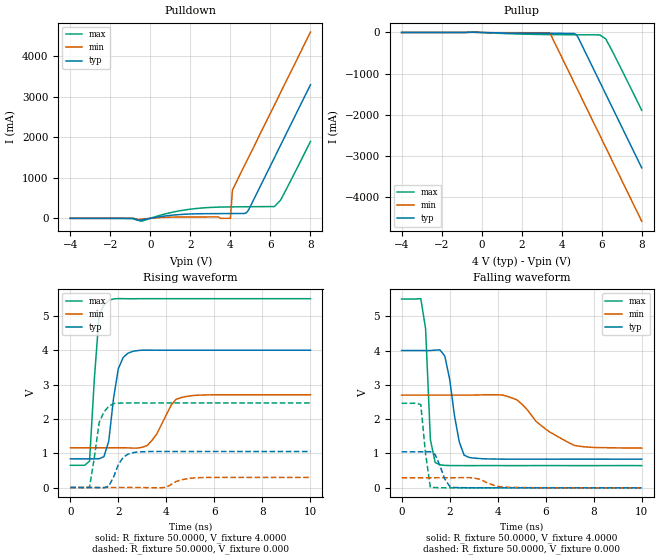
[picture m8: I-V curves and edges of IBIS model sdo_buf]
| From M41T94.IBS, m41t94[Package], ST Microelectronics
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|   Model sdo_buf
[Model]   sdo_buf
Model_type   Output
Polarity   Non-Inverting
Vmeas =   1.5000V
Cref =1.000e-10F
Rref =   0.6450k
Vref =   1.7300V
C_comp   7.8300pF   7.2500pF   8.5000pF
[Temperature Range]   27.0000   85.0000   -40.0000
[Voltage Range]   4.0000V   2.7000V   5.5000V
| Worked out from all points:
|   slope of the pulldown table from 0 to 0.6 V, typ, clamps not added: 12.4 ohm
|   slope of the pullup table from 0 to 0.6 V, typ, clamps not added: 80.2 ohm
|   rising waveform, R_fixture 50.0000, V_fixture 4.0000: 20-80 % time 359ps typ, 694ps min, 276ps max; typ from 0.835 V to 4 V
|   rising waveform, R_fixture 50.0000, V_fixture 0.000: 20-80 % time 434ps typ, 584ps min, 337ps max; typ from 0 V to 1.05 V
|   falling waveform, R_fixture 50.0000, V_fixture 4.0000: 20-80 % time 427ps typ, 1.5ns min, 180ps max; typ from 4 V to 0.835 V
|   falling waveform, R_fixture 50.0000, V_fixture 0.000: 20-80 % time 368ps typ, 636ps min, 238ps max; typ from 1.05 V to 0 V
[Pulldown]
| voltage   I(typ)   I(min)   I(max)
-4V       0A         0A         -600uA
-900mV    0A         0A         -7mA
-500mV    -45mA      -23.28mA   -72.71mA
1.6V      97.61mA    32.87mA    197mA
3.4V      116.6mA    33.89mA    276.6mA
4V        117.9mA    0A         281.9mA
4.1V      118.1mA    700mA      282.5mA
4.7V      120mA      1.3A       285.4mA
4.9V      202.4mA    1.5A       286.2mA
6.2V      1.5A       2.8A       291.2mA
6.5V      1.8A       3.1A       445.7mA
8V        3.3A       4.6A       1.899A
[Pullup]
| voltage   I(typ)   I(min)   I(max)
-4V       0A         0A         100uA
-400mV    5.701mA    2.743mA    10.5mA
3.4V      -21.56mA   -7.302mA   -51.47mA
4.6V      -23.5mA    -1.2A      -56.08mA
4.7V      -41.44mA   -1.3A      -56.35mA
4.8V      -103.4mA   -1.4A      -56.6mA
5.9V      -1.2A      -2.5A      -58.75mA
6.2V      -1.5A      -2.8A      -155.2mA
6.8V      -2.1A      -3.4A      -716.5mA
8V        -3.3A      -4.6A      -1.896A
[Ramp]
| variable   typ   min   max
dV/dt_r   2.1420/0.8210n   1.2358/2.1288n   3.1094/0.3905n
dV/dt_f   2.3600/0.2827n   1.5646/0.7749n   3.2700/0.1442n
R_load = 0.6450k
[Rising Waveform]
R_fixture = 50.0000
V_fixture = 4.0000
V_fixture_min = 2.7000
V_fixture_max = 5.5000
| time   V(typ)   V(min)   V(max)
0s        835.1mV    1.158V     647mV
800ps     835.2mV    1.158V     767.3mV
1ns       834.2mV    1.158V     3.169V
1.2ns     838.6mV    1.158V     5.023V
1.6ns     1.35V      1.158V     5.449V
2ns       3.465V     1.158V     5.503V
2.4ns     3.912V     1.155V     5.499V
3.2ns     4.002V     1.224V     5.5V
4.6ns     4V         2.617V     5.5V
10ns      4V         2.7V       5.5V
[Rising Waveform]
R_fixture = 50.0000
V_fixture = 0.000
V_fixture_min = 0.000
V_fixture_max = 0.000
| time   V(typ)   V(min)   V(max)
0s        741.4pV    876.5pV    598.6pV
800ps     -13.2uV    2.057uV    11.42mV
1.2ns     -3.072mV   -157.4nV   1.895V
1.6ns     40.49mV    -5.031uV   2.364V
1.8ns     304.2mV    -6.54uV    2.446V
2.2ns     878.6mV    83.83uV    2.461V
2.8ns     1.036V     -383uV     2.463V
4ns       1.049V     12.49mV    2.463V
5.2ns     1.048V     281mV      2.462V
10ns      1.048V     294mV      2.462V
[Falling Waveform]
R_fixture = 50.0000
V_fixture = 4.0000
V_fixture_min = 2.7000
V_fixture_max = 5.5000
| time   V(typ)   V(min)   V(max)
0s        4V         2.7V       5.5V
800ps     4V         2.7V       5.512V
1ns       4V         2.7V       4.635V
1.2ns     4V         2.7V       1.401V
1.4ns     4.01V      2.7V       735.9mV
1.8ns     3.837V     2.7V       653mV
2.6ns     954.7mV    2.7V       646.9mV
4.8ns     834.7mV    2.564V     646.7mV
7.2ns     835.2mV    1.234V     646.9mV
10ns      834.9mV    1.159V     646.8mV
[Falling Waveform]
R_fixture = 50.0000
V_fixture = 0.000
V_fixture_min = 0.000
V_fixture_max = 0.000
| time   V(typ)   V(min)   V(max)
0s        1.048V     293.9mV    2.462V
800ps     1.049V     293.9mV    2.425V
1ns       1.05V      294mV      978.9mV
1.2ns     1.052V     294.2mV    13.31mV
1.4ns     966.1mV    294.3mV    7.082mV
1.8ns     258mV      294.3mV    701.8uV
2ns       45.69mV    294.2mV    260.4uV
2.2ns     8.695mV    294.3mV    -28.41uV
4.4ns     -173.6uV   16.19mV    -4.79uV
10ns      236.1uV    18.59uV    -14.36uV
